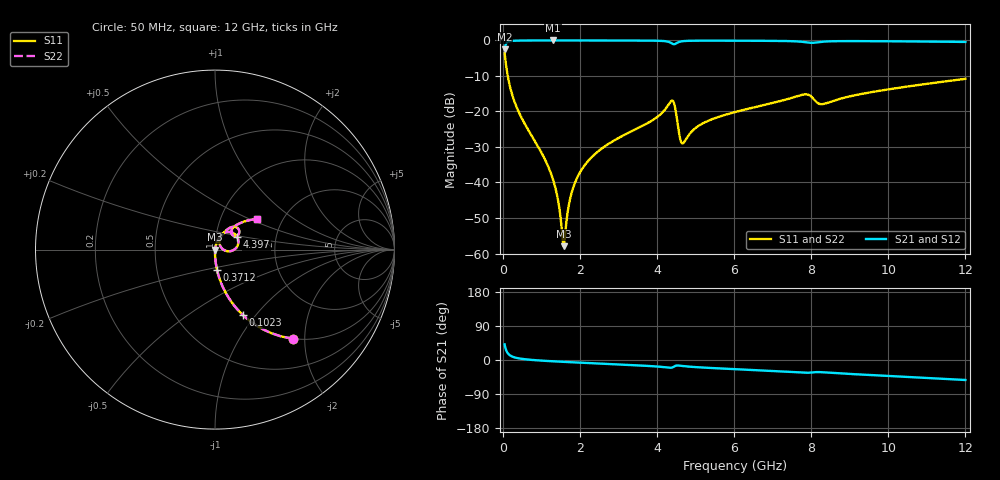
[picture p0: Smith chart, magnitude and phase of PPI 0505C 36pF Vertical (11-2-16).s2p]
# GHz S MA R 50
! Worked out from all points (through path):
!   1601 points, 50 MHz to 12 GHz, reference 50 ohm
!   highest |S21| = -0.01 dB at 1.305 GHz (marker M1); lowest = -2.5 dB at 50 MHz (marker M2)
!   group delay of S21, straight-line fit = 13 ps
!   lowest |S11| = -57.9 dB at 1.581 GHz (marker M3), VSWR 1.00, Z = 50.1 - j0.0142 ohm
!   |S11| at or under -10 dB: 131.4 MHz to end of sweep
!   |S22| runs from -57.9 to -3.6 dB; largest |S21 - S12| = 0
!   S11 on the Smith chart (normalised r, x): 50 MHz: 1.00, -1.76; 102.3 MHz: 1.00, -0.86; 371.2 MHz: 1.00, -0.22; 4.397 GHz: 1.27, +0.18; 12 GHz: 1.48, +0.55
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0.05  0.661 -48.8  0.7501 41.2  0.7501 41.2  0.661 -48.8
0.1022813  0.3944 -67.0  0.9185 22.9  0.9185 22.9  0.3944 -67.0
0.1844375  0.2295 -77.2  0.9728 12.7  0.9728 12.7  0.2295 -77.2
0.3711563  0.1116 -84.4  0.9931 5.3  0.9931 5.3  0.1116 -84.4
1.30475  0.01102 -87.4  0.9987 -3.4  0.9987 -3.4  0.01102 -87.4
1.42425  0.006088 -82.6  0.9987 -4.1  0.9987 -4.1  0.006088 -82.6
1.54375  0.001875 -52.7  0.9986 -4.7  0.9986 -4.7  0.001875 -52.7
1.581094  0.00127 -6.4  0.9986 -4.9  0.9986 -4.9  0.00127 -6.4
1.78275  0.006994 73.0  0.9985 -5.9  0.9985 -5.9  0.006994 73.0
2.044156  0.01507 77.3  0.9983 -7.2  0.9983 -7.2  0.01507 77.3
2.634187  0.03186 76.9  0.9976 -10.0  0.9976 -10.0  0.03186 76.9
4.038312  0.08593 67.6  0.9885 -17.4  0.9885 -17.4  0.08593 67.6
4.396813  0.1423 29.6  0.9013 -19.8  0.9013 -19.8  0.1423 29.6
4.4715  0.1134 2.4  0.8913 -15.9  0.8913 -15.9  0.1134 2.4
4.605937  0.04049 7.5  0.9622 -15.1  0.9622 -15.1  0.04049 7.5
4.673156  0.03557 32.7  0.9759 -16.0  0.9759 -16.0  0.03557 32.7
5.143688  0.06588 65.4  0.9918 -19.6  0.9918 -19.6  0.06588 65.4
6.025  0.09793 63.6  0.991 -24.2  0.991 -24.2  0.09793 63.6
8.019156  0.1589 33.4  0.9248 -32.9  0.9248 -32.9  0.1589 33.4
8.302969  0.1269 42.7  0.9592 -32.4  0.9592 -32.4  0.1269 42.7
10.01331  0.205 46.3  0.9727 -42.2  0.9727 -42.2  0.205 46.3
12  0.2878 36.2  0.9518 -52.8  0.9518 -52.8  0.2878 36.2
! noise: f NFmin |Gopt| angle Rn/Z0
0.05  0.0003948  0.8667  0.6749  0.0006367
1.372  0.004076  0.6802  4.301  0.002463
2.701  0.006961  0.6407  8.188  0.003642
4.031  0.01722  0.7674  12.3  0.0149
5.36  0.01585  0.6818  16.21  0.00946
6.682  0.0173  0.6466  19.84  0.009018
8.012  0.07285  0.8855  24.41  0.132
9.341  0.02519  0.6628  27.49  0.01352
10.67  0.02385  0.6104  30.53  0.01061
12  0.02555  0.599  33.68  0.01081
